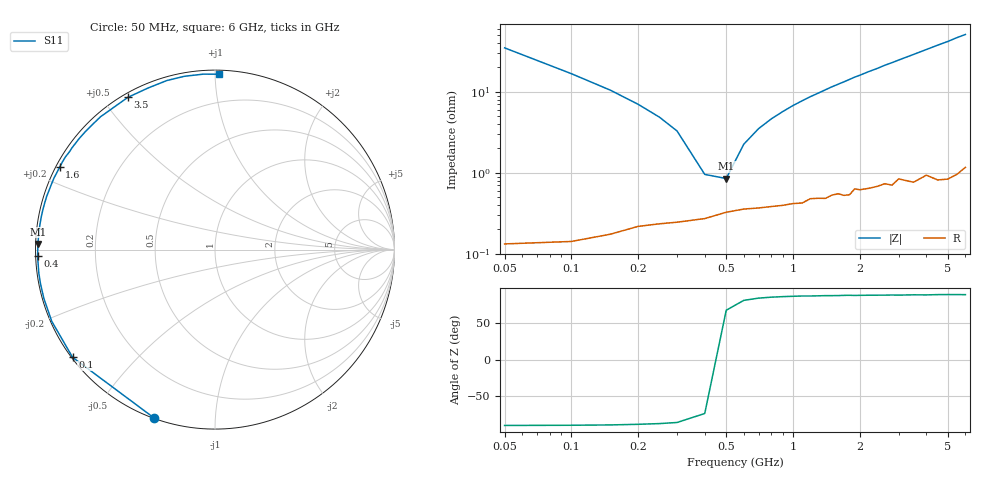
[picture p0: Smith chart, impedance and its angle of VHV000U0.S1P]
! Infineon Technologies  Discrete & RF Semiconductors
! BB 814
! Si Tuning Diode in SOT23
! VR = 0 V
! S-Parameters:  July  1999
# GHz  S  MA  R  50
!  f  S11
! GHz  MAG  ANG
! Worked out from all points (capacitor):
!   34 points, 50 MHz to 6 GHz, reference 50 ohm
!   read as one part to ground: C = 90.1 pF near 50 MHz
!   lowest |Z| = 850 mohm at 500 MHz (marker M1)
!   series resonance near 453.8 MHz, so ESL is about 1.4 nH
!   S11 on the Smith chart (normalised r, x): 50 MHz: 0.00, -0.70; 100 MHz: 0.00, -0.34; 400 MHz: 0.01, -0.02; 1.6 GHz: 0.01, +0.25; 3.5 GHz: 0.02, +0.58; 6 GHz: 0.02, +1.02
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0.05  0.9964 -110.1
0.1  0.9949 -142.9
0.15  0.9933 -156.3
0.2  0.9915 -164.0
0.25  0.9908 -168.9
0.3  0.9903 -172.5
0.4  0.9892 -177.9
0.5  0.987 178.2
0.6  0.9859 174.9
0.7  0.9855 172.0
0.8  0.9849 169.4
1  0.9838 164.6
1.2  0.9816 160.2
1.4  0.9817 156.1
1.6  0.9794 152.1
1.8  0.9804 148.2
1.9  0.9771 146.2
2.2  0.9774 140.8
2.4  0.9766 137.5
2.6  0.9755 133.8
2.8  0.977 130.7
3  0.9733 127.4
3.5  0.9774 119.8
4  0.9745 112.6
4.5  0.9794 105.9
5  0.9805 100.0
5.5  0.9798 93.8
6  0.9774 88.7
